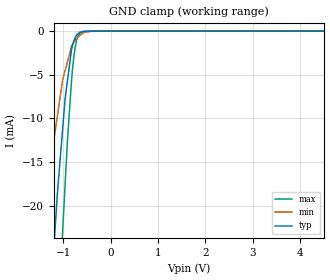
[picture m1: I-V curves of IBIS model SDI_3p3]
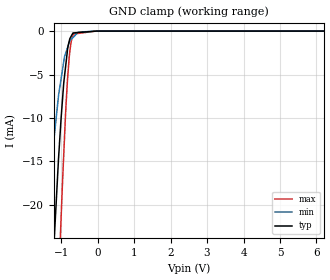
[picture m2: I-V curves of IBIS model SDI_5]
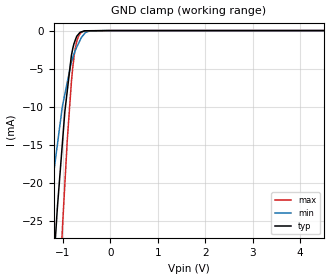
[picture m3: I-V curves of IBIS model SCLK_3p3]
|Texas Instruments Incorporated
|8/12-Bit, 1MSPS, 4-Channel, Bipolar Pseudo-Differential Low Power SAR
|   Analog-to-Digital Converter with Software-Selectable Ranges
| Marketing part#   Digital Voltage Range   Package-type   #pins
|ADS8634SRGER   2.7 to 5.25   QFN   24
|ADS8634SRGET   2.7 to 5.25   QFN   24
|ADS8638SRGER   2.7 to 5.25   QFN   24
|ADS8638SRGET   2.7 to 5.25   QFN   24
[IBIS Ver]   4.0
[File name]   ads8634_8.ibs
[File Rev]   1.0
[Date]   05/26/2011
[Source]   Texas Instruments Incorporated.
   Analog-eLab, HPA
   12500 TI Blvd
   Dallas, TX -75243
   For Support e-mail: elab_ibis@list.ti.com
[Notes]   Revision History:
   1.0: 04/14/2011
   - Initial version of the model
   - Initial Model generated from simulations in TISPICED
   - Model names with a trailing _3p3 contains the model for
   3.3V (3.0V and 3.6V).
   _ Model names with trailing _5 contains
   the model for 5V (4.75V and 5.25V) operation.
   - Model not matched to measurements
   - C_comp although listed in numerical order of value are
   obtained from varying PVT conditions. For PVT conditions
   for each specific value refer the buffer description under
   respective [Model]. IBIS model user is responsible for using
   appropriate C_comp to simulate for Signal Integrity.
   - Ignore warnings related to non-monotonicity as they are from
   TISPICE simulations
   2.0: 05/26/2011
   - Added ADS8634 product to this file and changed name from
   ads8648.ibs to ads8634_8.ibs
[Disclaimer]
  This model is designed as an aid for customers of Texas Instruments.
  TI and its licensors and suppliers make no warranties, either expressed
  or implied, with respect to this model, including the warranties of
  merchantability or fitness for a particular purpose.  The model is
  provided solely on an "as is" basis.  The entire risk as to its quality
  and performance is with the customer.
[Copyright] (C) Copyright 2011 Texas Instruments Incorporated.
   All rights reserved.
|   ADS8634 and ADS8638
[Component]   ads8634
[Manufacturer] TI
[Package]   | 24 pin, 4x4 QFN - PW package
| variable   typ   min   max
R_pkg  3.99618E-02   2.30000E-04   5.01500E-02
L_pkg  8.96061E-01nH 5.33000E-02nH 1.11386E+00nH
C_pkg  1.08525E-01pF 4.51000E-02pF 1.40050E-01pF
|-------------------------PIN------------------------------------------------
[Pin] signal_name  model_name  R_pin  L_pin C_pin
1   AVDD   POWER   0.02255  0.70471nH  0.13677pF
2   AGND   GND   0.01473  0.61466nH  0.15325pF
3   AGND   GND   0.00023  0.05330nH  0.04511pF
4   NC   NC   0.00023  0.05330nH  0.04510pF
5   AINCOM   TERM   0.04290  0.93148nH  0.10548pF
6   AIN7   TERM   0.05015  1.11386nH  0.11223pF
7   AIN6   TERM   0.04917  1.08816nH  0.11247pF
8   AIN5   TERM   0.04334  0.94018nH  0.11038pF
9   AIN4   TERM   0.04023  0.86340nH  0.10403pF
10  AIN3   TERM   0.04023  0.86135nH  0.10397pF
11  AIN2   TERM   0.04334  0.93478nH  0.11022pF
12  AIN1   TERM   0.04917  1.08047nH  0.11229pF
13  AIN0   TERM   0.05015  1.10356nH  0.11260pF
14  HVDD   POWER   0.02239  0.68551nH  0.14005pF
15  HVSS   GND   0.04543  0.98332nH  0.11179pF
16  _CS   SCLK   0.04328  0.93069nH  0.10676pF
17  SCLK   SCLK   0.04440  0.95873nH  0.11090pF
18  SDI   SDI   0.04953  1.08956nH  0.11232pF
19  SDO   SDO   0.04792  1.05222nH  0.10783pF
20  DGND   GND   0.03984  0.85333nH  0.10105pF
21  DVDD   POWER   0.03982  0.85247nH  0.10188pF
22  AL_PD   GPIO   0.04142  0.89253nH  0.10463pF
23  REFGND   GND   0.02011  0.59523nH  0.13294pF
24  REF   TERM   0.02150  0.65325nH  0.13367pF
[Component]   ads8638
[Manufacturer] TI
[Package]   | 24 pin, 4x4 QFN - PW package
| variable   typ   min   max
R_pkg  3.99618E-02   2.30000E-04   5.01500E-02
L_pkg  8.96061E-01nH 5.33000E-02nH 1.11386E+00nH
C_pkg  1.08525E-01pF 4.51000E-02pF 1.40050E-01pF
|-------------------------PIN------------------------------------------------
[Pin] signal_name  model_name  R_pin  L_pin C_pin
1   AVDD   POWER   0.02255  0.70471nH  0.13677pF
2   AGND   GND   0.01473  0.61466nH  0.15325pF
3   AGND   GND   0.00023  0.05330nH  0.04511pF
4   NC   NC   0.00023  0.05330nH  0.04510pF
5   AINCOM   TERM   0.04290  0.93148nH  0.10548pF
6   AIN7   TERM   0.05015  1.11386nH  0.11223pF
7   AIN6   TERM   0.04917  1.08816nH  0.11247pF
8   AIN5   TERM   0.04334  0.94018nH  0.11038pF
9   AIN4   TERM   0.04023  0.86340nH  0.10403pF
10  AIN3   TERM   0.04023  0.86135nH  0.10397pF
11  AIN2   TERM   0.04334  0.93478nH  0.11022pF
12  AIN1   TERM   0.04917  1.08047nH  0.11229pF
13  AIN0   TERM   0.05015  1.10356nH  0.11260pF
14  HVDD   POWER   0.02239  0.68551nH  0.14005pF
15  HVSS   GND   0.04543  0.98332nH  0.11179pF
16  _CS   SCLK   0.04328  0.93069nH  0.10676pF
17  SCLK   SCLK   0.04440  0.95873nH  0.11090pF
18  SDI   SDI   0.04953  1.08956nH  0.11232pF
19  SDO   SDO   0.04792  1.05222nH  0.10783pF
20  DGND   GND   0.03984  0.85333nH  0.10105pF
21  DVDD   POWER   0.03982  0.85247nH  0.10188pF
22  AL_PD   GPIO   0.04142  0.89253nH  0.10463pF
23  REFGND   GND   0.02011  0.59523nH  0.13294pF
24  REF   TERM   0.02150  0.65325nH  0.13367pF
|   Model Selectors
[Model Selector]  SDI
SDI_3p3   3.3V digital input
SDI_5   5V digital input
|NOTES   Model SDI split into two Models SDI_3p3 and SDI_5
|   to accomodate vast voltage range of 2.7V - 5.25V
|   SDI_3p3 operates in voltage range of 3 - 3.3 - 3.6
|   SDI_5 operates in voltage range of 4.75 - 5 - 5.25
|   The max pin frequency for Model SDI is 10MHz.Also the
|   voltage range and frequency is referenced with datasheet.
[Model Selector]  SCLK
SCLK_3p3   3.3V digital input
SCLK_5   5V digital input
|NOTES   Model SCLK split into two Models SCLK_3p3 and SCLK_5
|   to accomodate vast voltage range of 2.7V - 5.25V
|   SCLK_3p3 operates in voltage range of 3 - 3.3 - 3.6
|   SCLK_5 operates in voltage range of 4.75 - 5 - 5.25
|   The max pin frequency for Model SCLK is 20MHz.Also the
|   voltage range and frequency is referenced with datasheet.
[Model Selector]  GPIO
GPIO_3p3   3.3V digital I/O
GPIO_5   5V digital I/O
|NOTES   Model GPIO split into two Models GPIO_3p3 and GPIO_5
|   to accomodate vast voltage range of 2.7V - 5.25V
|   GPIO_3p3 operates in voltage range of 3 - 3.3 - 3.6
|   GPIO_5 operates in voltage range of 4.75 - 5 - 5.25
|   The max pin frequency for Model GPIO is 20MHz.Also the
|   voltage range and frequency is referenced with datasheet.
[Model Selector]  SDO
SDO_3p3  3.3V digital 3-state
SDO_5   5V digital 3-state
|NOTES   Model DOU split into two Models DOU_3p3 and DOU_5
|   to accomodate vast voltage range of 2.7V - 5.25V
|   DOU_3p3 operates in voltage range of 3 - 3.3 - 3.6
|   DOU_5 operates in voltage range of 4.75 - 5 - 5.25
|   The max pin frequency for Model DOU is 10MHz.Also the
|   voltage range and frequency is referenced with datasheet.
[Model Selector]  TERM
TERM_3p3  3.3V digital 3-state
TERM_5   5V digital 3-state
|   3.3V TERM Model
[Model] TERM_3p3
Model_type Terminator
C_comp   1e-20   1e-20   1e-20
| variable   typ   min   max
[Voltage Range]   3.3V   2.0V   5.5V
[POWER Clamp Reference]  3.3V   2.0V   5.5V
[GND Clamp Reference]   0.0V   0.0V   0.0V
|Operating Temperature   27   125   -40
[Temperature Range]   27   125   -40
|   5 V TERM Model
[Model] TERM_5
Model_type Terminator
C_comp   1e-20   1e-20   1e-20
| variable   typ   min   max
[Voltage Range]   5   4.75   5.25
[POWER Clamp Reference]   5   4.75   5.25
[GND Clamp Reference]   0.0V   0.0V   0.0V
|Operating Temperature   27   125   -40
[Temperature Range]   27   125   -40
| Models and submodels in the file (10): SDI_3p3 (Input), SDI_5 (Input), SCLK_3p3 (Input), SCLK_5 (Input), GPIO_3p3 (I/O), GPIO_5 (I/O), SDO_3p3 (3-state), SDO_5 (3-state), TERM_3p3 (Terminator), TERM_5 (Terminator)
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|NOTES   Model TERM split into two Models TERM_3p3 and TERM_5
|   to accomodate vast voltage range of 2.7V - 5.25V
|   TERM_3p3 operates in voltage range of 3 - 3.3 - 3.6
|   TERM_5 operates in voltage range of 4.75 - 5 - 5.25
|   The max pin frequency for Model TERM is 10MHz.Also the
|   voltage range and frequency is referenced with datasheet.
|   SDI_3p3   3.3V digital input Model
[Model] SDI_3p3  | 3.3V digital input
Model_type Input
Vinl = 0.99
Vinh = 2.31
|   typ   min   max
|   (nom PVT)   (Fast PVT)   (slow PVT)
|C_comp from L-C Tank method(L=1nH)
|Resonant Frequency(Hz)  4.41G   4.61G   4.18G
C_comp   1.30641E-12   1.19146E-12   1.45238E-12
| Where   nom PVT is  Nominal Process, 3.3V, 25C
|   Fast PVT is Strong Process, 3.6V, -40C
|   Slow PVT is Weak Process, 3.0V, 85C
|C_comp - from L-C Tank method, L = 1nH, peak frequency
[Model Spec]   | 3.3V
Vinl   0.99   0.9   1.08
Vinh   2.31   2.1   2.52
|Vinl = 0.3 DVDD
|Vinh = 0.7 DVDD
[Voltage Range]   3.3   3   3.6
[Temperature Range]   27   125   -40
[Power Clamp Reference]   3.3   3   3.6
[GND Clamp Reference]   0   0   0
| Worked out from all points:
|   GND clamp passes 1 mA (typ) near -0.77 V on its own axis
[GND Clamp]
|   Voltage   I(typ)   I(min)   I(max)
-3.3V     -249.3mA   -159.3mA   -320.6mA
-1.48V    -50.01mA   -26.11mA   -80.52mA
-1.342V   -36.96mA   -19.3mA    -62.4mA
-1.218V   -26.41mA   -13.19mA   -47.36mA
-1.129V   -18.95mA   -9.878mA   -36.61mA
-1.012V   -11.13mA   -5.547mA   -22.76mA
-961.2mV  -7.722mA   -4.509mA   -17.53mA
-914.5mV  -5.782mA   -3.565mA   -12.77mA
-827.1mV  -2.151mA   -1.797mA   -5.715mA
-751.3mV  -761.3uA   -1.053mA   -1.941mA
-658.1mV  -155.4uA   -517.8uA   -311.8uA
6.59V     0A         0A         0A
[POWER Clamp]
|   SCR cell for ESD function. Effects occurr above VDD x 2
|   Voltage   I(typ)   I(min)   I(max)
-3.3V     0A         0A         0A
0V        0A         0A         0A
6.6V      0A         0A         0A
|   SDI_5   5V digital input Model
[Model] SDI_5   | 5V digital input
Model_type Input
Vinl = 1.5
Vinh = 3.5
|   typ   min   max
|   (nom PVT)   (Fast PVT)   (slow PVT)
|C_comp from L-C Tank method(L=1nH)
|Resonant Frequency(Hz)  4.42G   4.74G   4.21G
C_comp   1.29444E-12   1.12741E-12   1.43245E-12
| Where   nom PVT is  Nominal Process, 5V, 25C
|   Fast PVT is Strong Process, 4.5V, -40C
|   Slow PVT is Weak Process, 5.5V, 85C
|C_comp - from L-C Tank method, L = 1nH, peak frequency
[Model Spec]   | 5V
Vinl   1.5   1.35   1.65
Vinh   3.5   3.15   3.85
|Vinl = 0.3 DVDD
|Vinh = 0.7 DVDD
[Voltage Range]   5   4.75   5.25
[Temperature Range]   27   125   -40
[Power Clamp Reference]   5   4.75   5.25
[GND Clamp Reference]   0   0   0
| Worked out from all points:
|   GND clamp passes 1 mA (typ) near -0.77 V on its own axis
[GND Clamp]
|   Voltage   I(typ)   I(min)   I(max)
-5V       -443.2mA   -304.1mA   -544.6mA
-1.434V   -45.47mA   -23.72mA   -74.19mA
-1.242V   -28.16mA   -14.26mA   -49.84mA
-1.074V   -14.88mA   -7.54mA    -29.73mA
-1.032V   -12.07mA   -6.331mA   -24.8mA
-1.001V   -10.04mA   -5.49mA    -21.52mA
-886.1mV  -4.416mA   -2.676mA   -10.23mA
-826.1mV  -2.209mA   -1.925mA   -5.649mA
-765.6mV  -957.7uA   -1.168mA   -2.458mA
-675.3mV  -214.5uA   -745.5uA   -512.7uA
-27.7mV   -870.2nA   0A         0A
9.985V    0A         0A         0A
|DVDD = 5V
[POWER Clamp]
|   SCR cell for ESD function. Effects occurr above VDD x 2
|   Voltage   I(typ)   I(min)   I(max)
-5V       0A         0A         0A
0V        0A         0A         0A
10V       0A         0A         0A
|   SCLK_3p3   3.3V digital input Model
[Model] SCLK_3p3   | 3.3V digital input
Model_type Input
Vinl = 0.99
Vinh = 2.31
|   typ   min   max
|   (nom PVT)   (Fast PVT)   (slow PVT)
|C_comp from L-C Tank method(L=1nH)
|Resonant Frequency(Hz)  3.91G   4.19G   3.81G
C_comp   1.65989E-12   1.44571E-12   1.74615E-12
| Where   nom PVT is  Nominal Process, 3.3V, 25C
|   Fast PVT is Strong Process, 3.6V, -40C
|   Slow PVT is Weak Process, 3.0V, 85C
|C_comp - from L-C Tank method, L = 1nH, peak frequency
[Model Spec]   | 3.3V
Vinl   0.99   0.9   1.08
Vinh   2.31   2.1   2.52
|Vinl = 0.3 DVDD
|Vinh = 0.7 DVDD
[Voltage Range]   3.3   3   3.6
[Temperature Range]   27   125   -40
[Power Clamp Reference]   3.3   3   3.6
[GND Clamp Reference]   0   0   0
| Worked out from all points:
|   GND clamp passes 1 mA (typ) near -0.73 V on its own axis
[GND Clamp]
|   Voltage   I(typ)   I(min)   I(max)
-3.3V     -287.8mA   -189.2mA   -371.8mA
-1.326V   -43.58mA   -26.23mA   -69.49mA
-1.218V   -33mA      -19.77mA   -54.48mA
-1.125V   -23.83mA   -15.29mA   -41.51mA
-1.018V   -15.19mA   -10.17mA   -26.68mA
-961.5mV  -10.68mA   -8.374mA   -20.24mA
-910.3mV  -7.945mA   -6.808mA   -14.45mA
-822.3mV  -3.272mA   -4.124mA   -6.711mA
-742.8mV  -1.284mA   -2.662mA   -2.402mA
-641.5mV  -235.6uA   -1.283mA   -431.9uA
-435.2mV  -21.07uA   -31.4uA    -43.36uA
6.59V     0A         0A         0A
[POWER Clamp]
|   SCR cell for ESD function. Effects occurr above VDD x 2
|   Voltage   I(typ)   I(min)   I(max)
-3.3V     0A         0A         0A
0V        0A         0A         0A
6.6V      0A         0A         0A
